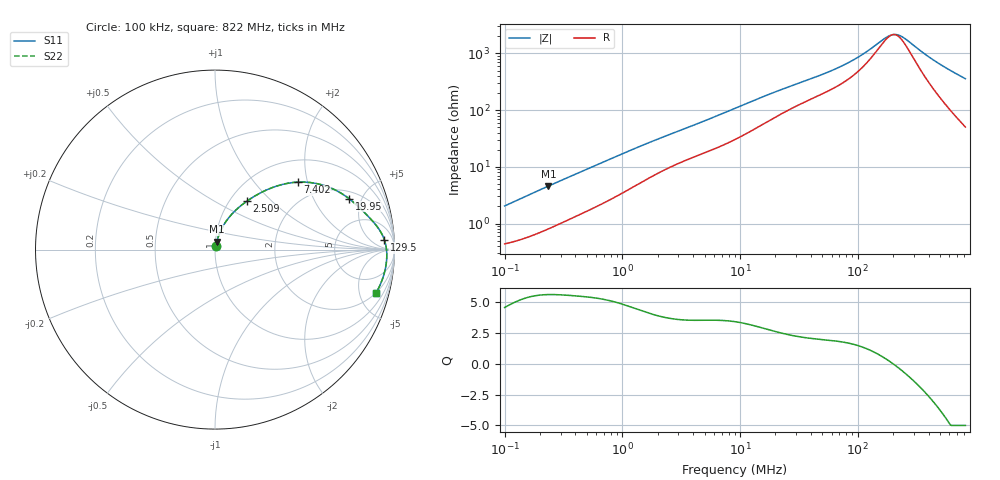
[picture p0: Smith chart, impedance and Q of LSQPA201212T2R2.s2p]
! LSQPA201212T2R2  S-PARAMETER MODEL  ( General Type )
! Model Generated by TAIYO YUDEN Corporation (http://www.ty-top.com)
! Version 2.0
! TAIYO YUDEN Control No. 100810NF25SB-FKC
! Copyright(c) 2007 TAIYO YUDEN CO.,LTD. All Rights Reserved.
! Product Description (link to TY-COMPAS)
! https://ds.yuden.co.jp/TYCOMPAS/or/detail?pn=LSQPA201212T2R2M&u=M
! Products Name : Inductors
! Characteristics :
!  Inductance : 2.2 uH , SRF(min) : 70 MHz , DC Resistance(max) : 0.429 Ohm
!  Rated Current : Saturation :530 mA , Temp Rise : 640 mA (40 degC)
!  Case Size : 2.0 x 1.25 / 0.079 x 0.049 [mm/inch] , Thickness : 1.25 / 0.049 [mm/inch]
!  (Conditions: Temperature = 25 degC , DC Bias Current/Voltage = 0A / 0V)
! External Node Assignments :
!  1  o---GGG---o  2
! GND o---------o GND
! Frequency Range : 0.1MHz  -  821.96004MHz  [ 402 STEP ]
# MHz S RI R 50
! Freq[MHz].  S11 Real  S11 Imag  S21 Real  S21 Imag  S12 Real  S12 Imag  S22 Real  S22 Imag
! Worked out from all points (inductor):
!   401 points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, 100 kHz to 822 MHz, reference 50 ohm
!   read as one part in series: L = 3.15 uH near 104.6 kHz
!   highest Q = 5.61 at 235.5 kHz (marker M1), where L = 3.05 uH
!   self-resonance near 199.7 MHz
!   S11 on the Smith chart (normalised r, x): 100 kHz: 1.01, +0.04; 2.509 MHz: 1.19, +0.72; 7.402 MHz: 1.50, +1.74; 19.95 MHz: 2.50, +3.93; 129.5 MHz: 18, +18; 822 MHz: 2.01, -7.09
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0.1  0.00474 0.0197  0.9953 -0.0197  0.9953 -0.0197  0.00474 0.0197
0.235457  0.00995 0.0443  0.9901 -0.0443  0.9901 -0.0443  0.00995 0.0443
0.452624  0.0211 0.0788  0.9789 -0.0788  0.9789 -0.0788  0.0211 0.0788
1.041984  0.0608 0.1563  0.9392 -0.1563  0.9392 -0.1563  0.0608 0.1563
2.048684  0.1414 0.2425  0.8586 -0.2425  0.8586 -0.2425  0.1414 0.2425
2.509338  0.1762 0.2689  0.8238 -0.2689  0.8238 -0.2689  0.1762 0.2689
4.309731  0.2953 0.3359  0.7047 -0.3359  0.7047 -0.3359  0.2953 0.3359
7.401866  0.4603 0.3757  0.5397 -0.3757  0.5397 -0.3757  0.4603 0.3757
9.272834  0.5368 0.3728  0.4632 -0.3728  0.4632 -0.3728  0.5368 0.3728
13.91172  0.6626 0.3357  0.3374 -0.3357  0.3374 -0.3357  0.6626 0.3357
19.95146  0.747 0.2838  0.253 -0.2838  0.253 -0.2838  0.747 0.2838
41.03579  0.8514 0.1873  0.1486 -0.1873  0.1486 -0.1873  0.8514 0.1873
58.85141  0.8888 0.1466  0.1112 -0.1466  0.1112 -0.1466  0.8888 0.1466
78.88411  0.9142 0.1131  0.0858 -0.1131  0.0858 -0.1131  0.9142 0.1131
101.076  0.9312 0.0838  0.0688 -0.0838  0.0688 -0.0838  0.9312 0.0838
129.5109  0.9438 0.0538  0.0562 -0.0538  0.0562 -0.0538  0.9438 0.0538
185.7378  0.9544 0.00919  0.0456 -0.00919  0.0456 -0.00919  0.9544 0.00919
207.8911  0.9561 -0.0051  0.0439 0.0051  0.0439 0.0051  0.9561 -0.0051
237.99  0.9571 -0.0226  0.0429 0.0226  0.0429 0.0226  0.9571 -0.0226
447.2994  0.9471 -0.1161  0.0529 0.1161  0.0529 0.1161  0.9471 -0.1161
627.1987  0.9273 -0.1795  0.0727 0.1795  0.0727 0.1795  0.9273 -0.1795
821.96  0.8987 -0.2391  0.1013 0.2391  0.1013 0.2391  0.8987 -0.2391
